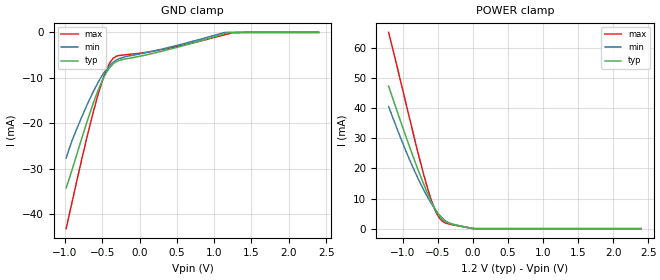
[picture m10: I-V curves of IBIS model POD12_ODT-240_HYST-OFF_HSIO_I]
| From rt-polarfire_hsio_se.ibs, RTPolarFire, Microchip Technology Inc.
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|   Model POD12_ODT-240_HYST-OFF_HSIO_I
[Model]   POD12_ODT-240_HYST-OFF_HSIO_I
Model_type   Input
Vinl =   0.76
Vinh =   0.92
|   typ   min   max
C_comp_pullup   1.335e-12   1.335e-12   1.380e-12
C_comp_pulldown  1.335e-12   1.335e-12   1.380e-12
[Temperature Range]  25C   125C   -55C
[Voltage Range]  1.2   1.14   1.26
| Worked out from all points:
|   POWER clamp passes 1 mA (typ) near -0.20 V on its own axis
[GND Clamp]
| Voltage   I(typ)   I(min)   I(max)
-984.4mV  -34.26mA   -27.71mA   -43.24mA
-866.2mV  -28.21mA   -22.22mA   -34.52mA
-708.7mV  -19.88mA   -16.13mA   -23.32mA
-590.6mV  -14.23mA   -12.07mA   -15.7mA
-472.5mV  -9.682mA   -8.769mA   -9.412mA
-393.7mV  -7.61mA    -7.174mA   -6.552mA
-354.4mV  -6.925mA   -6.583mA   -5.718mA
-315mV    -6.464mA   -6.126mA   -5.283mA
-196.9mV  -5.868mA   -5.366mA   -4.944mA
375mV     -3.824mA   -3.375mA   -3.527mA
1.2V      486.4nA    0A         -265.4uA
2.4V      0A         0A         0A
[POWER Clamp]
| Voltage   I(typ)   I(min)   I(max)
-1.2V     47.38mA    40.57mA    65.24mA
-1.063V   37.94mA    32.17mA    52.25mA
-905.6mV  27.45mA    23.15mA    37.03mA
-787.5mV  20mA       17.01mA    25.82mA
-669.4mV  13.06mA    11.54mA    15.39mA
-590.6mV  8.929mA    8.343mA    9.409mA
-551.3mV  7.099mA    6.9mA      6.92mA
-472.5mV  4.126mA    4.422mA    3.397mA
-433.1mV  3.081mA    3.44mA     2.436mA
-315mV    1.626mA    1.699mA    1.414mA
0V        0A         43.72uA    80.09uA
2.4V      0A         0A         0A
